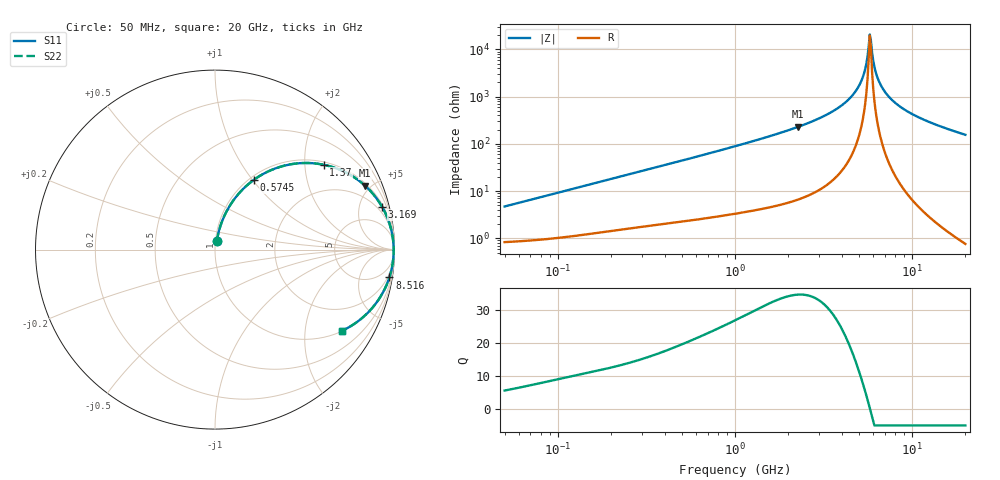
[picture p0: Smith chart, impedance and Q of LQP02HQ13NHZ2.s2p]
!Murata Part Number: LQP02HQ13NHZ2
!These Parameters are Measured in Series Mode Connection
!  o--[Z]--o
!Port1  Port2
!  o-------o
!Freq. Start=50[MHz] Stop=20[GHz], 401[Steps]
# Hz S RI R 50
!Freq.(Hz) S11(Real) S11(Imag) S21(Real) S21(Imag) S12(Real) S12(Imag) S22(Real) S22(Imag)
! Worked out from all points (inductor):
!   401 points, 50 MHz to 20 GHz, reference 50 ohm
!   read as one part in series: L = 14.8 nH near 51.52 MHz
!   highest Q = 34.7 at 2.279 GHz (marker M1), where L = 16.1 nH
!   self-resonance near 5.769 GHz
!   S11 on the Smith chart (normalised r, x): 50 MHz: 1.02, +0.09; 574.5 MHz: 1.05, +1.01; 1.37 GHz: 1.08, +2.50; 3.169 GHz: 1.24, +7.73; 8.516 GHz: 1, -12; 20 GHz: 1.02, -3.12
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5e7  0.0103 0.0457  0.9897 -0.0457  0.9897 -0.0457  0.0103 0.0457
1.364002e8  0.0263 0.1197  0.9737 -0.1197  0.9737 -0.1197  0.0263 0.1197
3.721004e8  0.1121 0.2872  0.8879 -0.2872  0.8879 -0.2872  0.1121 0.2872
5.745257e8  0.2157 0.3881  0.7843 -0.3881  0.7843 -0.3881  0.2157 0.3881
1e9  0.4449 0.4787  0.5551 -0.4787  0.5551 -0.4787  0.4449 0.4787
1.369645e9  0.6059 0.4726  0.3941 -0.4726  0.3941 -0.4726  0.6059 0.4726
2.279204e9  0.835 0.357  0.165 -0.357  0.165 -0.357  0.835 0.357
2.728004e9  0.893 0.2948  0.107 -0.2948  0.107 -0.2948  0.893 0.2948
3.168813e9  0.9307 0.2387  0.0693 -0.2387  0.0693 -0.2387  0.9307 0.2387
4.087748e9  0.9741 0.1391  0.0259 -0.1391  0.0259 -0.1391  0.9741 0.1391
4.81993e9  0.9893 0.0734  0.0107 -0.0734  0.0107 -0.0734  0.9893 0.0734
5.273168e9  0.9937 0.0374  0.00629 -0.0374  0.00629 -0.0374  0.9937 0.0374
5.433528e9  0.9946 0.0254  0.00542 -0.0254  0.00542 -0.0254  0.9946 0.0254
5.683258e9  0.9953 0.00741  0.00467 -0.00741  0.00467 -0.00741  0.9953 0.00741
5.769027e9  0.9954 0.0014  0.00457 -0.0014  0.00457 -0.0014  0.9954 0.0014
5.944466e9  0.9954 -0.0106  0.00459 0.0106  0.00459 0.0106  0.9954 -0.0106
6.125241e9  0.9951 -0.0226  0.00491 0.0226  0.00491 0.0226  0.9951 -0.0226
6.406762e9  0.9941 -0.0407  0.00594 0.0407  0.00594 0.0407  0.9941 -0.0407
7.442007e9  0.9857 -0.1009  0.0143 0.1009  0.0143 0.1009  0.9857 -0.1009
8.516016e9  0.9715 -0.1551  0.0285 0.1551  0.0285 0.1551  0.9715 -0.1551
1.220001e10  0.899 -0.2964  0.101 0.2964  0.101 0.2964  0.899 -0.2964
2e10  0.7077 -0.4524  0.2923 0.4524  0.2923 0.4524  0.7077 -0.4524
